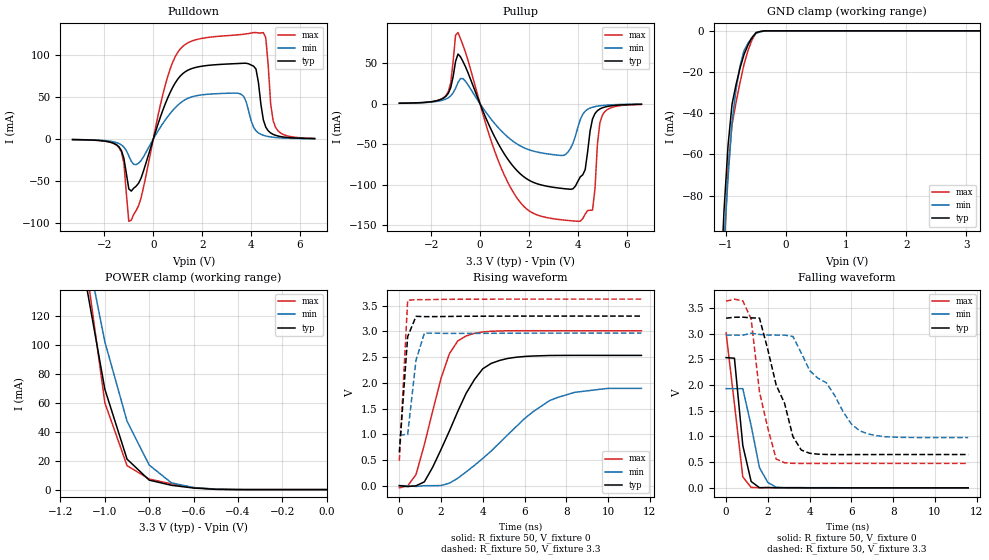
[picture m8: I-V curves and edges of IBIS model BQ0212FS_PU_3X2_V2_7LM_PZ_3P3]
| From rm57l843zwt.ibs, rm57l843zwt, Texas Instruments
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|   Model Cell PD_3X2_V2_7LM_PZ_3P3
|BQ0212FS_PU_3X2_V2_7LM_PZ_3P3
[Model]   BQ0212FS_PU_3X2_V2_7LM_PZ_3P3
Model_type   I/O
Polarity   Non-Inverting
Enable   Active-Low
Vinl =  1.25
Vinh =  1.65
Cref =  15.0001pF
Rref =  101.0000M
Vref =  0V
Vmeas =  1.65
C_comp   1.2p   1.2p   1.2p
[Model Spec]
Vinl   1.25   1.12   1.38
Vinh   1.65   1.45   1.75
[Temperature Range]   25   155   -40
[Voltage Range]   3.3   2.97   3.63
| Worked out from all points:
|   slope of the pulldown table from 0 to 0.495 V, typ, clamps not added: 11.8 ohm
|   slope of the pullup table from 0 to 0.495 V, typ, clamps not added: 14.3 ohm
|   GND clamp passes 1 mA (typ) near -0.50 V on its own axis
|   POWER clamp passes 1 mA (typ) near -0.59 V on its own axis
|   rising waveform, R_fixture 50, V_fixture 0: 20-80 % time 1.77ns typ, 3.13ns min, 1.22ns max; typ from 0 V to 2.54 V
|   rising waveform, R_fixture 50, V_fixture 3.3: 20-80 % time 283ps typ, 393ps min, 242ps max; typ from 0.648 V to 3.3 V
|   falling waveform, R_fixture 50, V_fixture 0: 20-80 % time 465ps typ, 593ps min, 516ps max; typ from 2.53 V to 0 V
|   falling waveform, R_fixture 50, V_fixture 3.3: 20-80 % time 1.14ns typ, 2.11ns min, 755ps max; typ from 3.3 V to 0.648 V
[POWER_clamp]
|   voltage   I(typ)   I(min)   I(max)
-3.3V     2.375A     2.63A      3.153A
-1.1V     156mA      180.2mA    173.4mA
-1.067V   127.2mA    154.3mA    135.6mA
-1.033V   98.41mA    128.4mA    97.92mA
-1V       69.61mA    102.5mA    60.2mA
-900mV    21.12mA    47.41mA    16.6mA
-800mV    6.574mA    17mA       7.307mA
-700mV    2.998mA    4.687mA    3.989mA
-600mV    1.086mA    1.404mA    1.425mA
-500mV    187uA      358uA      203.4uA
0V        430.3pA    12.78nA    319.6pA
[Pulldown]
|   voltage   I(typ)   I(min)   I(max)
-3.3V     -560.7uA   -504.5uA   -563.6uA
-1.4V     -9.199mA   -5.273mA   -10.11mA
-1.2V     -22.91mA   -9.491mA   -28.67mA
-1V       -59mA      -19.85mA   -97.49mA
-900mV    -61.64mA   -26.24mA   -96.13mA
1V        71.11mA    40.13mA    102.9mA
3.5V      89.74mA    54.24mA    123.8mA
4.2V      83.16mA    9.923mA    126.4mA
4.6V      14.26mA    3.714mA    120.5mA
4.8V      7.317mA    2.617mA    42.02mA
5V        4.531mA    1.939mA    13.99mA
6.6V      631.1uA    487.2uA    853.6uA
[Pullup]
|   voltage   I(typ)   I(min)   I(max)
-3.3V     614.6uA    591.9uA    551.1uA
-1.4V     9.028mA    5.738mA    10.01mA
-900mV    61.32mA    26.24mA    87.8mA
500mV     -34.85mA   -20.79mA   -49.88mA
1.4V      -78.76mA   -47.33mA   -111.2mA
3.4V      -104.6mA   -63.81mA   -143.4mA
4V        -95.71mA   -29.08mA   -145mA
4.3V      -81.25mA   -9.188mA   -136.1mA
4.6V      -18.8mA    -4.29mA    -131.2mA
4.8V      -8.576mA   -2.945mA   -49.93mA
5V        -5.064mA   -2.148mA   -14.33mA
6.6V      -672.1uA   -541.9uA   -866.9uA
[GND_clamp]
|   voltage   I(typ)   I(min)   I(max)
-3.3V     -1.951A    -1.627A    -3.261A
-1.1V     -130.1mA   -138.8mA   -166.7mA
-1.033V   -87.45mA   -103.2mA   -108mA
-966.7mV  -55.98mA   -71.77mA   -67.59mA
-900mV    -35.7mA    -44.42mA   -45.59mA
-833.3mV  -26.15mA   -28.61mA   -34.91mA
-766.7mV  -18.08mA   -17mA      -25.14mA
-700mV    -11.5mA    -9.608mA   -16.25mA
-633.3mV  -6.833mA   -5.978mA   -9.491mA
-500mV    -870.8uA   -1.241mA   -1.002mA
-300mV    -1.792uA   -15.69uA   -875.3nA
3.233V    409.6pA    4.016uA    238.5pA
[Ramp]
| variable   typ   min   max
dV/dt_f   1.620322/1.104801n   1.21722/2.126456n   1.92525/0.7621232n
dV/dt_r   1.545326/1.792782n   1.178757/3.282057n   1.835332/1.194061n
R_load = 50
[Rising Waveform]
R_fixture = 50
V_fixture = 0
V_fixture_min = 0
V_fixture_max = 0
|   time   V(typ)   V(min)   V(max)
0s        -78.65uV   106.7uV    -43.61mV
800ps     -3.402mV   -17.04mV   216.4mV
1.2ns     73.52mV    -1.046mV   799.2mV
2ns       705mV      2.217mV    2.09V
2.4ns     1.064V     47.83mV    2.568V
2.8ns     1.444V     142.7mV    2.816V
4ns       2.275V     531.1mV    2.99V
4.8ns     2.436V     831.2mV    3.01V
7.2ns     2.533V     1.655V     3.015V
11.6ns    2.535V     1.893V     3.014V
[Rising Waveform]
R_fixture = 50
V_fixture = 3.3
V_fixture_min = 2.97
V_fixture_max = 3.63
|   time   V(typ)   V(min)   V(max)
0s        648.4mV    982.3mV    484mV
400ps     2.9V       997.6mV    3.608V
800ps     3.295V     2.443V     3.62V
1.2ns     3.289V     2.967V     3.619V
11.6ns    3.3V       2.97V      3.63V
[Falling Waveform]
R_fixture = 50
V_fixture = 0
V_fixture_min = 0
V_fixture_max = 0
|   time   V(typ)   V(min)   V(max)
0s        2.534V     1.93V      3.014V
400ps     2.522V     1.93V      1.631V
800ps     825.7mV    1.93V      212.8mV
1.2ns     123.9mV    1.21V      8.826mV
1.6ns     2.752mV    391.6mV    2.308mV
2ns       6.685mV    104.5mV    3.097mV
2.4ns     2.548mV    12.82mV    1.348mV
2.8ns     3.775mV    860.6uV    358.4uV
11.6ns    5.03nV     30.74uV    -4.1uV
[Falling Waveform]
R_fixture = 50
V_fixture = 3.3
V_fixture_min = 2.97
V_fixture_max = 3.63
|   time   V(typ)   V(min)   V(max)
0s        3.3V       2.97V      3.63V
800ps     3.32V      2.969V     3.638V
1.2ns     3.307V     3.007V     3.286V
1.6ns     3.301V     2.983V     1.864V
2.4ns     1.999V     2.972V     560.7mV
3.2ns     998.9mV    2.944V     477.4mV
4ns       673.5mV    2.283V     474.7mV
4.8ns     649.5mV    2.045V     475.4mV
6.4ns     647.4mV    1.111V     475.7mV
11.6ns    648.2mV    978.8mV    475.6mV
